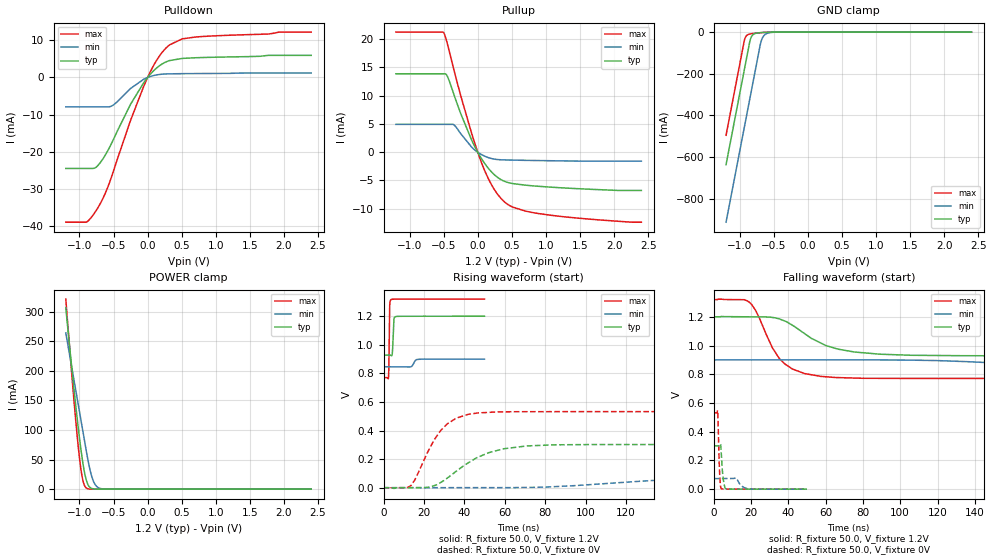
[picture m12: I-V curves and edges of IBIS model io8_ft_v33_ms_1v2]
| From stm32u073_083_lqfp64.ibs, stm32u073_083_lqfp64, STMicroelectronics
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[Model]   io8_ft_v33_ms_1v2
Model_type I/O
Polarity   Non-Inverting
Enable   Active-Low
| CAP_THRESHOLD on pad IOFT is "UDTCAPC" :
| Rising=30.0% of vddiom   Falling=70.0% of vddiom
| C_comp min and max val. don't necessarily correlate with the min and max pvt
| but are the smallest and greatest pad capacitance found.
| var   typ   min   max
C_comp   1.89804pF  1.82361pF  1.89871pF
|C_comp_pullup   1.10155pF  1.05685pF  1.08560pF
|C_comp_pulldown   796.49000fF  766.75501fF  813.11001fF
Vinl = 270.0mV
Vinh = 924.0mV
Vmeas = 600.0mV   | Reference voltage for timing measurements
Cref  = 50.0pF   | Timing specification test load capacitance value
Rref  = 100.0MOhm   | Timing specification test load resistance value
Vref  = 600.0mV   | Timing specification test load voltage
[Model Spec]
| TIME_THRESHOLD on pin ZIV33M is "CMOS" :
| Rising=50.0% of vddiom   Falling=50.0% of vddiom
Vinl 458.70000mV 364.70000mV 499.70000mV
Vinh 728.30000mV 548.30000mV 792.30000mV
| variable   typ   min   max
[Temperature Range] 25.0 140.0 -40.0
| variable   typ   min   max
[Voltage Range] 1.2V 900.0mV 1.32V
| variable   typ   min   max
[POWER Clamp Reference] 1.2V 900.0mV 1.32V
| variable   typ   min   max
[GND Clamp Reference] 0V 0V 0V
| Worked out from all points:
|   slope of the pulldown table from 0 to 0.18 V, typ, clamps not added: 55.6 ohm
|   slope of the pullup table from 0 to 0.18 V, typ, clamps not added: 56.3 ohm
|   GND clamp passes 1 mA (typ) near -0.61 V on its own axis
|   POWER clamp passes 1 mA (typ) near -0.81 V on its own axis
|   rising waveform, R_fixture 50.0, V_fixture 1.2V: 20-80 % time 436ps typ, 1.26ns min, 275ps max; typ from 0.928 V to 1.2 V
|   falling waveform, R_fixture 50.0, V_fixture 1.2V: 20-80 % time 23ns typ, 63.2ns min, 13.6ns max; typ from 1.2 V to 0.928 V
|   rising waveform, R_fixture 50.0, V_fixture 0V: 20-80 % time 20.6ns typ, 52.3ns min, 12.8ns max; typ from 0 V to 0.302 V
|   falling waveform, R_fixture 50.0, V_fixture 0V: 20-80 % time 1.14ns typ, 2.95ns min, 781ps max; typ from 0.302 V to 0 V
[POWER Clamp]
-1.2V     306.2mA    263.9mA    321.2mA
-1.09V    180mA      191mA      163.4mA
-1.05V    136.9mA    164.5mA    110.9mA
-1.01V    96.55mA    138mA      64.02mA
-960mV    52.29mA    104.9mA    20.68mA
-930mV    31.08mA    85.01mA    7.282mA
-900mV    15.67mA    65.13mA    2.025mA
-850mV    3.417mA    35.2mA     196.2uA
-800mV    570.2uA    14.97mA    18.13uA
-750mV    88.98uA    4.952mA    1.667uA
-680mV    6.495uA    823.9uA    58.96nA
2.4V      0A         0A         0A
[GND Clamp]
-1.2V     -636.9mA   -913.2mA   -495.8mA
-940mV    -194.9mA   -471.2mA   -53.78mA
-920mV    -160.9mA   -437.2mA   -28.06mA
-890mV    -109.9mA   -386.2mA   -14.28mA
-850mV    -43.09mA   -318.2mA   -9.18mA
-820mV    -18.33mA   -267.2mA   -7.516mA
-780mV    -7.695mA   -199.2mA   -5.87mA
-690mV    -2.548mA   -49.42mA   -2.9mA
-660mV    -1.868mA   -24.06mA   -2.112mA
-630mV    -1.326mA   -12.18mA   -1.447mA
-430mV    -19.32uA   -177.8uA   -8.091uA
2.4V      298.5pA    77.04nA    207.1pA
| variable   typ   min   max
[Pullup Reference] 1.2V 900.0mV 1.32V
| variable   typ   min   max
[Pulldown Reference] 0V 0V 0V
[Pullup]
-1.2V     13.87mA    4.927mA    21.25mA
-500mV    13.87mA    4.927mA    21.15mA
-450mV    13.53mA    4.927mA    19.38mA
-350mV    10.23mA    4.844mA    14.6mA
-90mV     2.161mA    908.5uA    3.352mA
40mV      -840.8uA   -309uA     -1.362mA
130mV     -2.46mA    -847.3uA   -4.016mA
230mV     -3.829mA   -1.199mA   -6.331mA
420mV     -5.274mA   -1.376mA   -9.06mA
510mV     -5.544mA   -1.401mA   -9.708mA
900mV     -6.043mA   -1.482mA   -10.87mA
2.4V      -6.768mA   -1.593mA   -12.38mA
[Pulldown]
-1.2V     -24.47mA   -7.9mA     -38.94mA
-890mV    -24.47mA   -7.9mA     -38.83mA
-720mV    -23.49mA   -7.9mA     -34.76mA
-610mV    -20.54mA   -7.9mA     -30.69mA
-510mV    -17.01mA   -7.49mA    -25.69mA
-250mV    -7.205mA   -2.955mA   -11.53mA
0V        -15fA      0A         0A
160mV     2.97mA     779.9uA    5.417mA
320mV     4.547mA    983.4uA    8.763mA
510mV     5.135mA    1.031mA    10.4mA
700mV     5.311mA    1.057mA    10.88mA
2.4V      5.965mA    1.209mA    12.22mA
[Ramp]
dV/dt_r 181.2704mV/20.57753ns 44.07287mV/52.2852ns 319.21358mV/12.7905ns
dV/dt_f 162.91944mV/22.98286ns 32.17702mV/63.12873ns 329.55738mV/13.62946ns
R_load = 50.0
| Removed startup time: 0s 0s 0s  .
| Removed end time: 49.9ns.
[Rising Waveform]
R_fixture   = 50.0
V_fixture   = 1.2V
V_fixture_min = 900.0mV
V_fixture_max = 1.32V
0s        928.4mV    846.4mV    770.7mV
2.4ns     928.6mV    846.4mV    771.5mV
2.6ns     928.6mV    846.4mV    869.5mV
2.9ns     928.6mV    846.4mV    1.226V
3ns       928.4mV    846.4mV    1.277V
3.6ns     925.4mV    846.4mV    1.316V
4.3ns     941.9mV    846.4mV    1.319V
5.1ns     1.18V      846.4mV    1.319V
5.8ns     1.197V     846.4mV    1.319V
49.9ns    1.2V       899.9mV    1.32V
| Removed startup time: 0s 0s 0s  .
| Removed end time: 399.9ns.
[Falling Waveform]
R_fixture   = 50.0
V_fixture   = 1.2V
V_fixture_min = 900.0mV
V_fixture_max = 1.32V
0s        1.2V       900mV      1.32V
18.8ns    1.2V       900.4mV    1.304V
22.3ns    1.2V       900.3mV    1.248V
35.1ns    1.186V     900mV      910.9mV
42.2ns    1.141V     900mV      836.3mV
56.9ns    1.021V     900mV      785.7mV
75.3ns    955.2mV    900mV      773.6mV
105.6ns   932.2mV    898.4mV    770.8mV
210.5ns   928.5mV    854mV      770.7mV
399.9ns   928.5mV    846.4mV    770.7mV
| Removed startup time: 0s 0s 0s  .
| Removed end time: 399.9ns.
[Rising Waveform]
R_fixture   = 50.0
V_fixture   = 0V
V_fixture_min = 0V
V_fixture_max = 0V
0s        -2.587uV   2.342uV    -6.107uV
13.5ns    -133.1uV   -219.6uV   14.53mV
24.8ns    13.08mV    -32.43uV   330.2mV
28.1ns    35.35mV    -31.36uV   398mV
35.8ns    113.7mV    -27.51uV   485.7mV
46.5ns    212.1mV    4.396uV    522.7mV
59.3ns    272.1mV    163.9uV    530.8mV
85ns      300mV      7.517mV    532mV
171.4ns   302.1mV    67.57mV    532mV
399.9ns   302.1mV    73.45mV    532mV
| Removed startup time: 0s 0s 0s  .
| Removed end time: 49.9ns.
[Falling Waveform]
R_fixture   = 50.0
V_fixture   = 0V
V_fixture_min = 0V
V_fixture_max = 0V
0s        302.1mV    73.45mV    532mV
2.1ns     301.9mV    73.45mV    545.6mV
3ns       301.9mV    73.46mV    149.7mV
3.5ns     314.1mV    73.46mV    34.89mV
3.9ns     277.7mV    73.46mV    3.785mV
5ns       78.47mV    73.46mV    1.141mV
6.6ns     1.537mV    73.42mV    388.2uV
11.9ns    145.5uV    77.5mV     239.4uV
18.5ns    120.4uV    1.681mV    257uV
49.9ns    59.51uV    28.33uV    3.207uV
